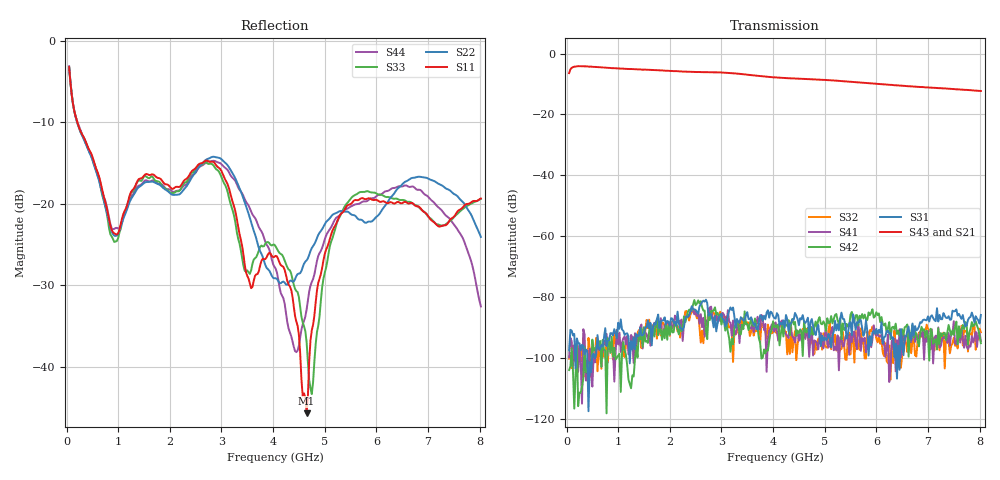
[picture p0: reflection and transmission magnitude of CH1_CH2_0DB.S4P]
!Agilent Technologies,E5071C,MY46316741,A.11.02
!Date: Thu May 28 14:23:46 2026
!Data & Calibration Information:
!1:CH1 INPUT 2:CH1 OUTPUT 3:CH2 INPUT 4:CH2 OUTPUT
!Freq	S11:SOLT4(ON)	S12:SOLT4(ON)	S13:SOLT4(ON)	S14:SOLT4(ON)
!	S21:SOLT4(ON)	S22:SOLT4(ON)	S23:SOLT4(ON)	S24:SOLT4(ON)
!	S31:SOLT4(ON)	S32:SOLT4(ON)	S33:SOLT4(ON)	S34:SOLT4(ON)
!	S41:SOLT4(ON)	S42:SOLT4(ON)	S43:SOLT4(ON)	S44:SOLT4(ON)
!PortZ  Port1:50+j0  Port2:50+j0  Port3:50+j0  Port4:50+j0
!Above PortZ is port z conversion or system Z0 setting when saving the data.
!When reading, reference impedance value at option line is always used.
# Hz S dB R 50
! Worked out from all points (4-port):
!   320 points, 50 MHz to 8.025 GHz, reference 50 ohm
!   strongest paths, dB at 50 MHz, 2.05 GHz, 4.05 GHz, 6.05 GHz, 8.025 GHz:
!     S43: -6.4, -5.7, -7.9, -10.0, -12.3
!     S21: -6.5, -5.9, -7.9, -10.0, -12.3
!     S31: -97.5, -87.1, -87.0, -90.7, -85.8
!     S42: -103.9, -91.6, -89.3, -85.3, -95.1
!     S41: -99.8, -90.1, -88.3, -92.9, -94.3
!     S32: -100.2, -88.1, -91.6, -92.4, -91.5
!   lowest |S11| = -45.7 dB at 4.65 GHz (marker M1), VSWR 1.01, Z = 49.6 - j0.273 ohm
!   |S11| at or under -10 dB: 209.2 MHz to end of sweep
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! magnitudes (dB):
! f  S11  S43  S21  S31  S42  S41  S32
! 50 MHz  -3.2  -6.4  -6.5  -97.5  -103.9  -99.8  -100.2
! 925 MHz  -23.6  -4.8  -4.9  -90.5  -96.6  -107.7  -91.2
! 2.85 GHz  -14.9  -6.2  -6.3  -89.9  -84.3  -86.9  -85.0
! 4.225 GHz  -28.1  -8.0  -8.1  -90.1  -88.5  -91.4  -91.3
! 4.65 GHz  -45.7  -8.4  -8.5  -87.8  -91.6  -91.4  -90.4
! 5.425 GHz  -20.3  -9.1  -9.2  -93.6  -88.8  -92.3  -100.6
! 8.025 GHz  -19.4  -12.3  -12.3  -85.8  -95.1  -94.3  -91.5
